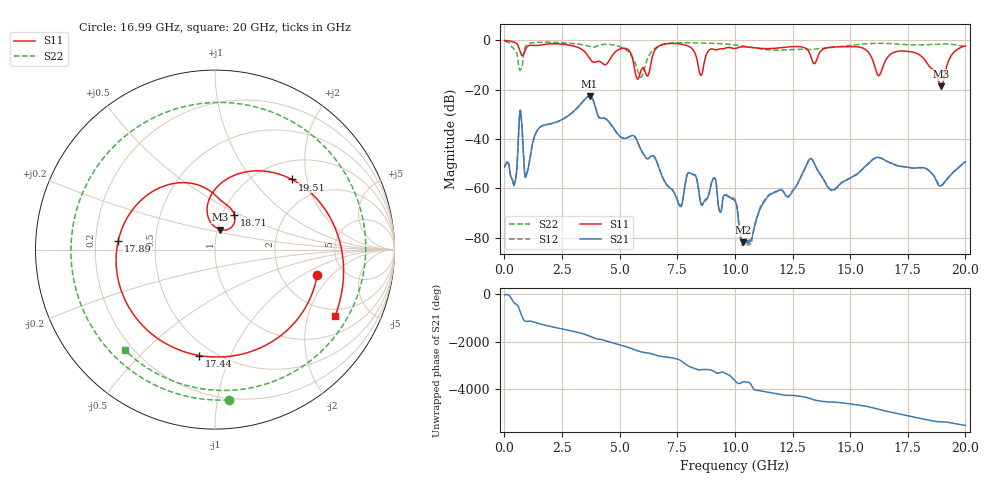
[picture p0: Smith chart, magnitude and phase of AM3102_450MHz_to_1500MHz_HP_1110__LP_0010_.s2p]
!Agilent Technologies,E8364B,MY43040894,A.07.50.67
!Agilent E8364B: A.07.50.67
!Date: Thursday, January 11, 2018 06:42:37
!Correction: S11(Full 2 Port(1,2))
!S21(Full 2 Port(1,2))
!S12(Full 2 Port(1,2))
!S22(Full 2 Port(1,2))
!S2P File: Measurements: S11, S21, S12, S22:
# Hz S  dB  R 50
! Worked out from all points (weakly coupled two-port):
!   1601 points, 10 MHz to 20 GHz, reference 50 ohm
!   highest |S21| = -22.65 dB at 3.696 GHz (marker M1); lowest = -82.0 dB at 10.34 GHz (marker M2)
!   lowest |S11| = -18.8 dB at 18.95 GHz (marker M3), VSWR 1.26, Z = 51.6 + j11.7 ohm
!   |S11| at or under -10 dB: 5.618 GHz to 6.347 GHz (729 MHz wide, 12.2 % of centre); 16.05 GHz to 16.45 GHz (401.7 MHz wide, 2.47 % of centre); 18.39 GHz to 19.21 GHz (821.9 MHz wide, 4.37 % of centre)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
!   |S22| runs from -15.0 to -0.4 dB; largest |S21 - S12| = 0.0034
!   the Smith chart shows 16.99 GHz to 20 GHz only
!   S11 on the Smith chart (normalised r, x): 16.99 GHz: 3.21, -1.36; 17.44 GHz: 0.42, -0.77; 17.89 GHz: 0.30, +0.04; 18.71 GHz: 1.14, +0.47; 19.51 GHz: 1.39, +1.63; 20 GHz: 1.68, -3.00
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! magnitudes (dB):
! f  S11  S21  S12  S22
! 10 MHz  -0.1  -51.5  -51.0  -0.4
! 447.3 MHz  -0.9  -57.8  -57.7  -3.9
! 697.2 MHz  -5.0  -28.5  -28.5  -12.1
! 959.5 MHz  -3.0  -54.6  -54.4  -1.9
! 1.484 GHz  -2.1  -35.8  -35.8  -0.9
! 3.346 GHz  -3.6  -25.5  -25.5  -1.8
! 3.696 GHz  -7.3  -22.6  -22.6  -2.5
! 5.92 GHz  -12.5  -44.4  -44.3  -15.0
! 6.682 GHz  -2.5  -51.1  -51.1  -2.4
! 7.619 GHz  -1.5  -67.4  -66.8  -1.0
! 10.01 GHz  -3.4  -65.2  -64.6  -1.9
! 10.34 GHz  -2.7  -82.0  -82.6  -2.3
! 13.34 GHz  -7.8  -48.2  -48.2  -3.8
! 14.23 GHz  -2.8  -60.7  -60.9  -2.9
! 16.68 GHz  -6.4  -49.5  -49.5  -1.3
! 16.99 GHz  -4.6  -50.7  -50.7  -1.5
! 17.44 GHz  -4.5  -51.4  -51.4  -1.8
! 17.89 GHz  -5.3  -51.8  -51.7  -1.9
! 18.71 GHz  -13.0  -56.4  -56.2  -1.6
! 18.95 GHz  -18.8  -58.9  -58.9  -1.5
! 19.51 GHz  -4.7  -53.2  -53.2  -1.8
! 20 GHz  -2.3  -49.3  -49.5  -2.5
